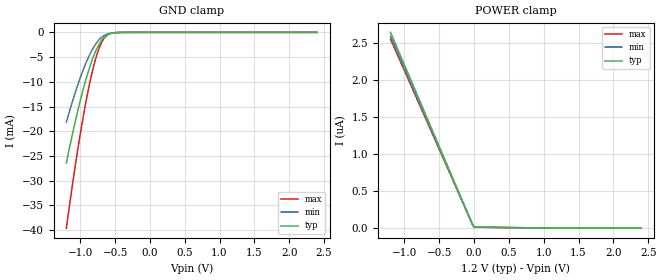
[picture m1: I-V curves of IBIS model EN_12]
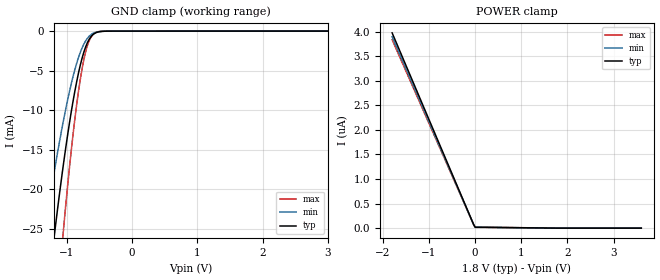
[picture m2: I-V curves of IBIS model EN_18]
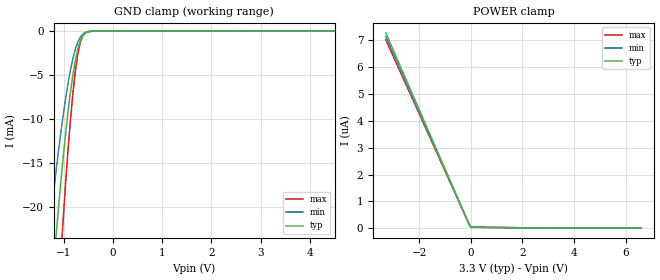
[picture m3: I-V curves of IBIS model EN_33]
| Texas Instruments Incorporated
| HDMI Companion Chip with Step-up converter, I2C Level Shifter
| Marketing part#   Voltage Range   Package-type   #pins/pkg drawing
| TPD5S115YFF   1.65V-5.5V   YFF   16-ball YFF
[IBIS Ver]   4.0
[File name]   tpd5s115.ibs
[File Rev]   1.0
[Date]   09/08/2012
[Source]   TIspiceD simulations
   Texas Instruments Incorporated.
   Analog eLab Design Center, HPA
   12500 TI Blvd
   Dallas, TX -75243
   For Support e-mail: elab_scm_ibis@list.ti.com
[Notes]   Revision History:
   Rev 1.0: 09/08/2012
   - C_comp although listed in numerical order of value are
   obtained from varying PVT conditions.
   For PVT conditions for each specific value, refer to the
   buffer description under respective [Model].
   IBIS model user is responsible for using appropriate
   C_comp to simulate for Signal Integrity.
   - IBIS model not matched to TISPICED simulations
   - non-monotonic behavior in power clamp and combined pullup/down
   waveforms is per simulations
   - internal weak pullup to 10kOhms is part of the characterisitcs
[Disclaimer] This model is designed as an aid for customers of Texas Instruments.
 TI and its licensors and suppliers make no warranties, either expressed
 or implied, with respect to this  model, including the warranties of
 merchantability or fitness for a particular purpose.
 The model is provided solely on an "as is" basis. The entire risk as to
 its quality and performance is with the customer.
[Copyright] (C)Copyright 2012 Texas Instruments Incorporated.
   All rights reserved.
|   Component TPD5S115YFF
[Component]   TPD5S115YFF
[Manufacturer]  Texas Instruments Incorporated
[Package]   |16-ball YFF
|   typ   min   max
R_pkg   0.005   0.004   0.006
L_pkg   0.20nH   0.196nH   0.25nH
C_pkg   0.65pF   0.533pF   0.652pF
[Pin]   signal_name   model_name   R_pin   L_pin   C_pin
A1   SCLB   DDCB_5  0.004   0.199nH   0.602pF
A2   GND   GND   0.005   0.205nH   0.573pF
A3   HPDB   HPDB_5  0.006   0.231nH   0.639pF
A4   VCCA   POWER   0.005   0.199nH   0.602pF
B1   CECB   CECB_5  0.005   0.199nH   0.602pF
B2   SDAB   DDCB_5  0.005   0.199nH   0.602pF
B3   LS_OE   EN   0.005   0.204nH   0.579pF
B4   HPDA   HPDA   0.006   0.226nH   0.608pF
C1   5VOUT   NC   0.005   0.236nH   0.652pF
C2   SW   NC   0.005   0.236nH   0.652pF
C3   EN   EN   0.005   0.199nH   0.602pF
C4   SDAA   DDCA   0.006   0.22nH   0.605pF
D1   PGND   GND   0.005   0.25nH   0.633pF
D2   VBAT   POWER   0.006   0.235nH   0.633pF
D3   CECA   CECA   0.005   0.186nH   0.533pF
D4   SCLA   DDCA   0.005   0.192nH   0.544pF
[Pin Mapping] pulldown_ref pullup_ref gnd_clamp_ref power_clamp_ref |ext_ref
A1   gndbus   NC   gndbus   vccabus
A2   gndbus   NC
A3   NC   NC   gndbus   vccabus
A4   NC   vccabus
B1   gndbus   NC   gndbus   vccabus
B2   gndbus   NC   gndbus   vccabus
B3   NC   NC   gndbus   vccabus
B4   gndbus   vccabus   gndbus   vccabus
C1   NC   NC
C2   NC   NC
C3   NC   NC   gndbus   vccabus
C4   gndbus   NC   gndbus   vccabus
D1   gndbus   NC
D2   NC   vccabus
D3   gndbus   NC   gndbus   vccabus
D4   gndbus   NC   gndbus   vccabus
[Model Selector] HPDA
HPDA_12 1.2V supply
HPDA_18 1.8V supply
HPDA_33 3.3V supply
[Model Selector] EN
EN_12 1.2V supply
EN_18 1.8V supply
EN_33 3.3V supply
[Model Selector] DDCA
DDCA_12 1.2V supply
DDCA_18 1.8V supply
DDCA_33 3.3V supply
[Model Selector] CECA
CECA_12 1.2V supply
CECA_18 1.8V supply
CECA_33 3.3V supply
| Models and submodels in the file (15): EN_12 (Input), EN_18 (Input), EN_33 (Input), HPDA_33 (I/O), HPDA_18 (I/O), HPDA_12 (I/O), CECA_12 (I/O_open_sink), CECA_18 (I/O_open_sink), CECA_33 (I/O_open_sink), DDCA_33 (I/O_open_sink), DDCA_12 (I/O_open_sink), DDCA_18 (I/O_open_sink), HPDB_5 (Input), DDCB_5 (I/O_open_sink), CECB_5 (I/O_open_sink)
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[Model]   EN_12
Model_type   Input
Vinl = 0.4V
Vinh = 1.0V
|   typ   min   max
C_comp   0.9916pF   0.9796pF   1.0277pF
[Voltage Range]   1.200V   1.100V   1.300V
|Junction temperature
[Temperature Range]   40.0   100.0   -40.0
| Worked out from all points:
|   GND clamp passes 1 mA (typ) near -0.66 V on its own axis
|ambient temperature   25   85   -40
[GND Clamp]
|   Voltage   I(typ)   I(min)   I(max)
-1.2V     -26.38mA   -18.14mA   -39.58mA
-1.11V    -20.37mA   -13.83mA   -30.52mA
-1.019V   -14.87mA   -9.926mA   -22.2mA
-946.7mV  -10.92mA   -7.157mA   -16.19mA
-874.4mV  -7.452mA   -4.777mA   -10.89mA
-802mV    -4.572mA   -2.864mA   -6.499mA
-747.7mV  -2.872mA   -1.777mA   -3.918mA
-693.5mV  -1.614mA   -999.3uA   -2.04mA
-621.1mV  -607.8uA   -390.4uA   -637uA
-548.7mV  -180.5uA   -128.7uA   -143.8uA
-422.1mV  -15.52uA   -15.34uA   -7.207uA
2.4V      2.662uA    2.374uA    2.761uA
[POWER Clamp]
|   Voltage   I(typ)   I(min)   I(max)
-1.2V     2.648uA    2.596uA    2.556uA
-24.12mV  53.23nA    52.17nA    51.37nA
0V        12.9nA     11.8nA     11.96nA
2.4V      0A         0A         0A
[Model]   EN_18
Model_type   Input
Vinl = 0.4V
Vinh = 1.0V
|   typ   min   max
C_comp   0.9536pF   0.9386pF   0.9995pF
[Voltage Range]   1.800V   1.650V   1.950V
|Junction temperature
[Temperature Range]   40.0   100.0   -40.0
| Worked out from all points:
|   GND clamp passes 1 mA (typ) near -0.66 V on its own axis
|ambient temperature   25   85   -40
[GND Clamp]
|   Voltage   I(typ)   I(min)   I(max)
-1.8V     -74.61mA   -53.05mA   -110.3mA
-1.339V   -36.42mA   -25.35mA   -54.56mA
-1.176V   -24.73mA   -16.95mA   -37.1mA
-1.067V   -17.73mA   -11.95mA   -26.54mA
-1.04V    -16.1mA    -10.8mA    -24.07mA
-931.7mV  -10.15mA   -6.627mA   -15.02mA
-850.3mV  -6.421mA   -4.083mA   -9.318mA
-796mV    -4.362mA   -2.728mA   -6.18mA
-714.6mV  -2.049mA   -1.266mA   -2.683mA
-606mV    -480.5uA   -313.4uA   -478.2uA
-416.1mV  -13.74uA   -13.82uA   -6.241uA
3.6V      3.992uA    3.561uA    4.142uA
[POWER Clamp]
|   Voltage   I(typ)   I(min)   I(max)
-1.8V     3.972uA    3.893uA    3.834uA
-36.18mV  79.84nA    78.26nA    77.06nA
0V        18.86nA    17.55nA    17.34nA
3.6V      0A         0A         0A
[Model]   EN_33
Model_type   Input
Vinl = 0.4V
Vinh = 1.0V
|   typ   min   max
C_comp   0.9070pF   0.8804pF   0.9723pF
[Voltage Range]   3.300V   3.000V   3.600V
|Junction temperature
[Temperature Range]   40.0   100.0   -40.0
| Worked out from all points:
|   GND clamp passes 1 mA (typ) near -0.65 V on its own axis
|ambient temperature   25   85   -40||
[GND Clamp]
|   Voltage   I(typ)   I(min)   I(max)
-3.3V     -1.126A    -863.3mA   -1.505A
-1.31V    -34.28mA   -23.81mA   -51.37mA
-1.26V    -30.64mA   -21.19mA   -45.95mA
-1.161V   -23.72mA   -16.23mA   -35.58mA
-1.111V   -20.46mA   -13.9mA    -30.67mA
-1.061V   -17.36mA   -11.69mA   -25.98mA
-1.012V   -14.44mA   -9.621mA   -21.54mA
-862.3mV  -6.928mA   -4.423mA   -10.09mA
-762.8mV  -3.301mA   -2.048mA   -4.568mA
-663.3mV  -1.107mA   -692uA     -1.312mA
-563.8mV  -236.3uA   -163.8uA   -200.2uA
6.6V      7.319uA    6.529uA    7.699uA
[POWER Clamp]
|   Voltage   I(typ)   I(min)   I(max)
-3.3V     7.283uA    7.14uA     7.028uA
-66.33mV  146.4nA    143.5nA    141.3nA
0V        34.24nA    33.68nA    33.3nA
6.6V      0A         0A         0A
